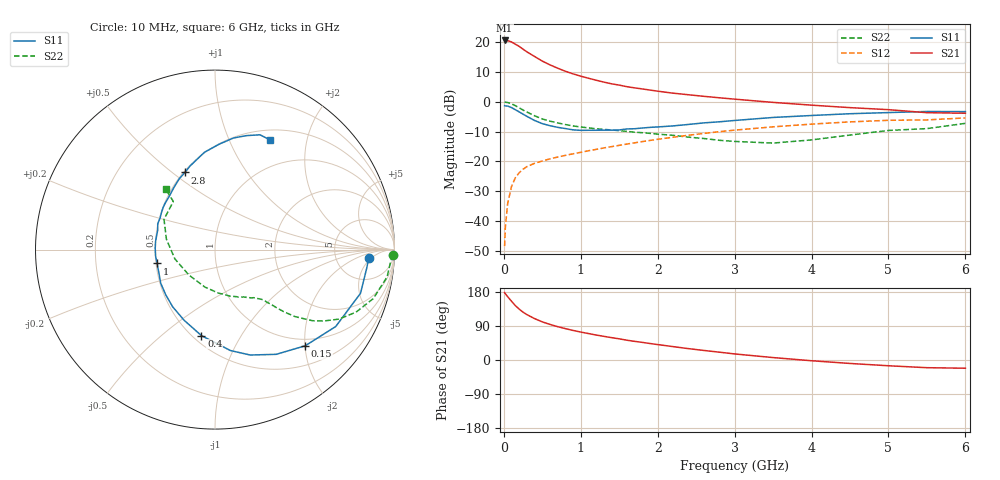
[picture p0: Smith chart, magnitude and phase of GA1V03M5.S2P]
! Infineon Technologies  Discrete & RF Semiconductors
! BF775
! Si NPN RF Bipolar Junction Transistor in SOT23
! VCE = 1 V  IC = 3.5 mA
! Common Emitter S-Parameters:  May  1996
# GHz  S  MA  R  50
!  f  S11  S21  S12  S22
! GHz  MAG  ANG  MAG  ANG  MAG  ANG  MAG  ANG
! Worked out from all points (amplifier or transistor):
!   36 points, 10 MHz to 6 GHz, reference 50 ohm
!   highest |S21| = 20.5 dB at 10 MHz (marker M1)
!   |S21| within 3 dB of that: start of sweep to 254.1 MHz
!   unconditionally stable (mu >= 1): 847 MHz to end of sweep
!   at 250 MHz: K = 0.41, MSG = 20.1 dB, |S12| = -22.6 dB
!   at 1.4 GHz: K = 1.18, MAG = 8.0 dB, |S12| = -15.1 dB
!   at 6 GHz: K = 1.04, MAG = -0.5 dB, |S12| = -5.4 dB
!   S11 on the Smith chart (normalised r, x): 10 MHz: 11, -4; 150 MHz: 0.86, -2.01; 400 MHz: 0.55, -0.69; 1 GHz: 0.51, -0.09; 2.8 GHz: 0.51, +0.56; 6 GHz: 0.62, +1.42
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0.01  0.8571 -3.3  10.65 177.7  0.0038 86.7  0.9921 -1.7
0.02  0.852 -6.8  10.5 174.7  0.008 84.7  0.9817 -3.6
0.05  0.8465 -16.7  10.57 167.0  0.0199 80.3  0.9711 -9.0
0.1  0.7976 -32.5  10.04 155.0  0.038 72.6  0.9232 -17.2
0.15  0.7349 -46.8  9.214 143.4  0.0533 65.2  0.8598 -23.9
0.2  0.6758 -59.7  8.466 134.2  0.0647 60.1  0.7915 -29.3
0.25  0.6194 -71.5  7.603 126.2  0.0739 55.8  0.7244 -33.3
0.3  0.569 -81.3  6.858 119.7  0.0819 53.0  0.6727 -36.1
0.4  0.4849 -99.0  5.728 109.2  0.093 49.4  0.5825 -39.9
0.5  0.43 -113.5  4.802 100.6  0.1018 47.6  0.5156 -42.1
0.6  0.3967 -126.4  4.146 93.9  0.1103 46.9  0.4731 -43.3
0.8  0.3556 -148.3  3.242 82.8  0.1263 46.6  0.4152 -45.2
1  0.3317 -166.5  2.684 73.7  0.1421 47.3  0.3777 -47.0
1.1  0.3328 -174.1  2.478 69.8  0.151 47.7  0.3647 -48.6
1.3  0.3342 172.2  2.134 62.4  0.1683 47.6  0.3437 -51.2
1.6  0.35 155.7  1.788 52.2  0.1956 47.1  0.3188 -56.6
2.2  0.3936 129.8  1.393 35.3  0.2544 44.1  0.2739 -71.7
2.8  0.4613 111.3  1.166 20.7  0.3151 38.5  0.226 -94.9
3.5  0.5454 96.2  0.976 6.4  0.3799 30.1  0.203 -135.7
4.5  0.6301 80.6  0.797 -9.1  0.4599 17.1  0.2766 168.0
5.5  0.687 68.6  0.656 -20.3  0.4965 3.1  0.3548 130.9
6  0.6836 63.6  0.642 -21.7  0.5358 -0.7  0.4346 129.2
